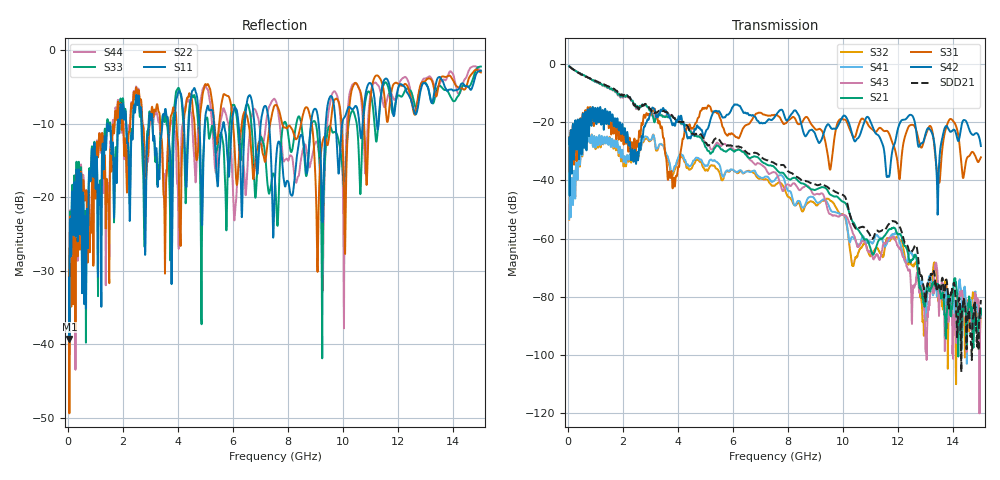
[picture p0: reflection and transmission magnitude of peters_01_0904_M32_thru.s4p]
# MHZ S RI R 50.00
! FREQ  S11  S12  S13  S14
!  S21  S22  S23  S24
!  S31  S32  S33  S34
!  S41  S42  S43  S44
!  REAL  IMAG  REAL  IMAG  REAL  IMAG  REAL  IMAG
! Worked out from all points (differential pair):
!   1496 points, 50 MHz to 15 GHz, reference 50 ohm
!   strongest paths, dB at 50 MHz, 3.79 GHz, 7.53 GHz, 11.27 GHz, 15 GHz:
!     S42: -25.4, -20.8, -18.1, -24.5, -28.3
!     S31: -25.3, -39.9, -17.6, -22.4, -32.1
!     S21: -0.8, -18.0, -35.8, -61.1, -84.1
!     S43: -0.8, -17.8, -37.3, -66.2, -84.3
!     S41: -53.4, -36.9, -39.8, -59.2, -84.1
!     S32: -53.5, -38.5, -41.7, -63.6, -87.2
!   taken as a pair (ports 1,3 in; 2,4 out), SDD21 dB: -0.9, -17.7, -34.3, -57.5, -81.1
!   lowest |S11| = -39.3 dB at 60 MHz (marker M1), VSWR 1.02, Z = 51 + j0.327 ohm
!   |S11| at or under -10 dB: start of sweep to 1.437 GHz; 1.451 GHz to 1.822 GHz (370.8 MHz wide, 22.7 % of centre); 7.31 GHz to 8.832 GHz (1.521 GHz wide, 18.9 % of centre)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
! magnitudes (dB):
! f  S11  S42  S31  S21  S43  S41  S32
! 50 MHz  -30.9  -25.4  -25.3  -0.8  -0.8  -53.4  -53.5
! 60 MHz  -39.3  -29.7  -29.3  -0.9  -0.9  -48.9  -48.9
! 3.09 GHz  -11.0  -15.1  -16.3  -18.1  -17.3  -24.6  -24.6
! 3.86 GHz  -10.8  -20.6  -39.7  -18.6  -18.5  -35.7  -37.0
! 5.12 GHz  -8.0  -21.4  -14.3  -29.9  -28.0  -33.8  -35.9
! 9.25 GHz  -23.4  -25.1  -23.4  -42.4  -44.6  -46.7  -47.0
! 15 GHz  -2.8  -28.3  -32.1  -84.1  -84.3  -84.1  -87.2
